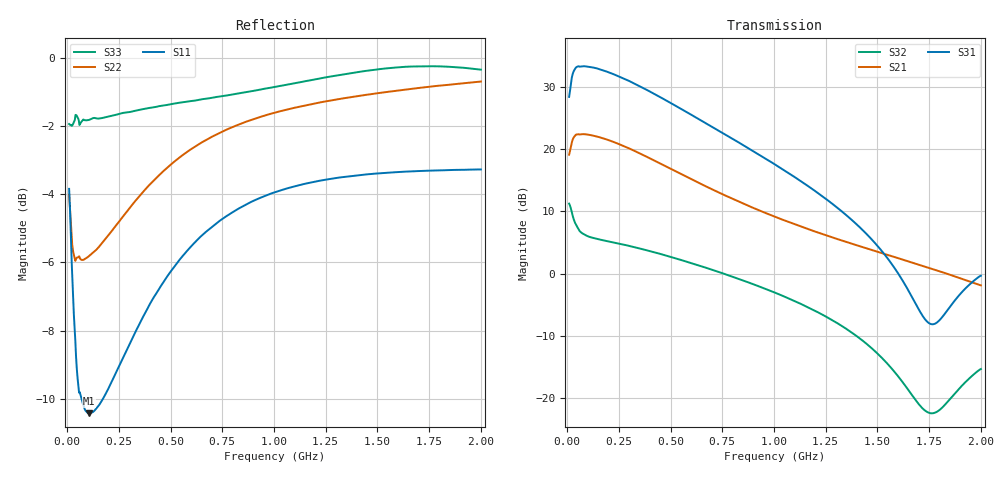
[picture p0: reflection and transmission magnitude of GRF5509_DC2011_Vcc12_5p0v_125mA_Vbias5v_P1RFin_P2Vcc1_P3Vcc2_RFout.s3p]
!Keysight Technologies,N5244B,MY57181157,A.18.40.03
!Date: Wednesday, April 29, 2026 14:24:33
!Correction: S11(C  3-Port  )
!S12(C  3-Port  )
!S13(C  3-Port  )
!S21(C  3-Port  )
!S22(C  3-Port  )
!S23(C  3-Port  )
!S31(C  3-Port  )
!S32(C  3-Port  )
!S33(C  3-Port  )
!S3P File: Measurements: <S11,S12,S13>,
!<S21,S22,S23>,
!<S31,S32,S33>:
# Hz S  dB  R 50
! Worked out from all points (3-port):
!   1991 points, 10 MHz to 2 GHz, reference 50 ohm
!   strongest paths, dB at 10 MHz, 507 MHz, 1.005 GHz, 1.503 GHz, 2 GHz:
!     S31: 28.3, 27.2, 17.5, 4.3, -0.3
!     S21: 19.1, 16.7, 9.1, 3.5, -1.9
!     S32: 11.2, 2.6, -3.1, -12.9, -15.3
!   lowest |S11| = -10.4 dB at 105 MHz (marker M1), VSWR 1.86, Z = 30.1 - j14.2 ohm
!   |S11| at or under -10 dB: 69.86 MHz to 173.9 MHz (104 MHz wide, 85.3 % of centre)
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1e7  -3.84 -55.0  -22.24 -35.0  -56.19 -94.1
     19.06 -137.3  -4.00 -79.5  -31.86 -84.0
     28.34 78.5  11.22 -173.2  -1.93 -111.7
3e7  -7.13 -92.4  -26.74 -42.8  -65.60 125.9
     21.70 -161.8  -5.70 -123.7  -42.42 148.6
     32.28 32.7  8.94 162.3  -1.92 -147.0
4.4e7  -8.82 -110.4  -28.78 -42.6  -64.31 -55.0
       22.29 -172.8  -5.89 -137.6  -41.99 -36.7
       33.08 16.5  7.80 158.6  -1.67 -157.7
1.05e8  -10.43 -134.5  -32.42 -31.6  -72.93 106.4
        22.26 163.5  -5.82 -157.7  -50.79 31.8
        33.17 -16.6  5.92 154.7  -1.81 -169.2
1.73e8  -10.01 -139.8  -33.43 -26.5  -70.66 79.9
        21.71 146.2  -5.41 -162.0  -45.39 43.9
        32.61 -38.9  5.34 148.1  -1.75 -171.9
2.54e8  -9.01 -141.1  -34.02 -25.5  -64.66 84.8
        20.73 129.2  -4.78 -164.1  -42.48 43.3
        31.58 -60.5  4.77 138.8  -1.63 -172.8
4.77e8  -6.47 -145.4  -35.31 -27.8  -61.68 82.5
        17.21 94.4  -3.25 -169.7  -39.78 32.0
        27.80 -107.2  2.90 113.3  -1.38 -173.0
6.68e8  -5.12 -150.9  -36.37 -29.2  -58.32 83.5
        14.04 74.6  -2.41 -174.8  -39.49 27.0
        24.18 -137.2  0.96 94.1  -1.19 -172.9
1.005e9  -3.94 -160.1  -37.75 -29.7  -55.11 86.5
         9.11 52.5  -1.60 178.1  -40.23 29.7
         17.50 -178.1  -3.07 65.1  -0.84 -173.2
2e9  -3.27 -178.9  -40.61 -42.6  -48.33 92.0
     -1.89 10.2  -0.69 156.3  -34.94 70.8
     -0.35 -126.5  -15.32 122.9  -0.34 172.1
